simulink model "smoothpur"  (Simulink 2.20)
settings: Solver=ode45  StartTime=0  StopTime=5.0  MaxStep=.01  RelTol=1e-3  AbsTol=1e-3
undefined symbols (not defined in the file or in its folder): sfuny

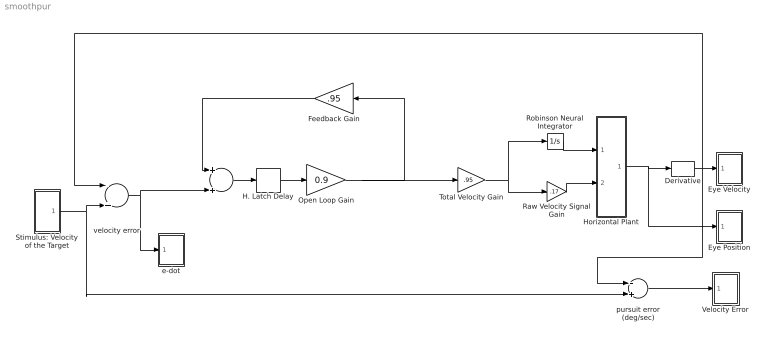
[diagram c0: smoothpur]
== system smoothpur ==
  "  " : Sum  Inputs=++
  Derivative : Derivative
  Eye Position : Subsystem  LoadFcn=sfuny([],[],[],'LoadBlock')  StartFcn=sfuny([],[],[],'Start')  StopFcn=sfuny([],[],[],'Stop')  mask(Graph scope.){}
      mask help: Graph scope using MATLAB graph window. Enter plotting ranges and line type.
      mask init:
      | color = @4; ax = [0, @1, @2, @3]; dt = -1;
  Eye Velocity : Subsystem  LoadFcn=sfuny([],[],[],'LoadBlock')  StartFcn=sfuny([],[],[],'Start')  StopFcn=sfuny([],[],[],'Stop')  mask(Graph scope.){}
      mask help: Graph scope using MATLAB graph window. Enter plotting ranges and line type.
      mask init:
      | color = @4; ax = [0, @1, @2, @3]; dt = -1;
  Feedback Gain : Gain  Orientation=left  Gain=.95
  H. Latch Delay : TransportDelay  DelayTime=.07  InitialInput=00  BufferSize=1024
  Horizontal Plant : Subsystem
  Open Loop Gain : Gain  Gain=0.9
  Raw Velocity Signal Gain : Gain  Gain=.17
  Robinson Neural Integrator : Integrator  ExternalReset=none  InitialConditionSource=internal  InitialCondition=0  LimitOutput=off  UpperSaturationLimit=inf  LowerSaturationLimit=-inf  ShowSaturationPort=off  ShowStatePort=off  AbsoluteTolerance=auto
  Stimulus: Velocity of the Target : Subsystem
  Total Velocity Gain : Gain  Gain=.95
  Velocity Error : Subsystem  LoadFcn=sfuny([],[],[],'LoadBlock')  StartFcn=sfuny([],[],[],'Start')  StopFcn=sfuny([],[],[],'Stop')  mask(Graph scope.){}
      mask help: Graph scope using MATLAB graph window. Enter plotting ranges and line type.
      mask init:
      | color = @4; ax = [0, @1, @2, @3]; dt = -1;
  e-dot : Subsystem  LoadFcn=sfuny([],[],[],'LoadBlock')  StartFcn=sfuny([],[],[],'Start')  StopFcn=sfuny([],[],[],'Stop')  mask(Graph scope.){}
      mask help: Graph scope using MATLAB graph window. Enter plotting ranges and line type.
      mask init:
      | color = @4; ax = [0, @1, @2, @3]; dt = -1;
  pursuit error (deg/sec) : Sum  Inputs=-+
  velocity error : Sum  Inputs=-+
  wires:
  Raw Velocity Signal Gain/1 -> Horizontal Plant/2(in_2)
  Robinson Neural Integrator/1 -> Horizontal Plant/1(in_1)
  Horizontal Plant/1(out_1) -> Derivative/1, Eye Position/1(x)
  Feedback Gain/1 -> "  "/1
  Stimulus: Velocity of the Target/1(out_1) -> velocity error/2, pursuit error (deg/sec)/2
  pursuit error (deg/sec)/1 -> Velocity Error/1(x)
  Derivative/1 -> pursuit error (deg/sec)/1, Eye Velocity/1(x), velocity error/1
  Open Loop Gain/1 -> Feedback Gain/1, Total Velocity Gain/1
  Total Velocity Gain/1 -> Robinson Neural Integrator/1, Raw Velocity Signal Gain/1
  "  "/1 -> H. Latch Delay/1
  H. Latch Delay/1 -> Open Loop Gain/1
  velocity error/1 -> e-dot/1(x), "  "/2

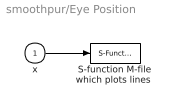
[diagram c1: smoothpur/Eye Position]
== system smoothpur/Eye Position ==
  x : Inport  Port=1  PortWidth=-1  SampleTime=-1
  "S-function M-file which plots lines " : S-Function  FunctionName=sfuny  Parameters=ax, color,dt  PortCounts=[]  SFunctionModules=''
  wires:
  x/1 -> "S-function M-file which plots lines "/1

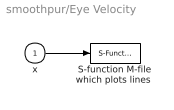
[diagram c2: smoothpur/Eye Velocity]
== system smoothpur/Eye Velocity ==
  x : Inport  Port=1  PortWidth=-1  SampleTime=-1
  "S-function M-file which plots lines " : S-Function  FunctionName=sfuny  Parameters=ax, color,dt  PortCounts=[]  SFunctionModules=''
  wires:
  x/1 -> "S-function M-file which plots lines "/1

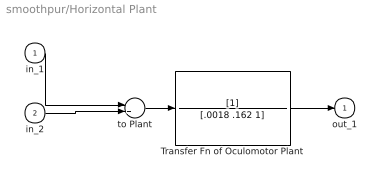
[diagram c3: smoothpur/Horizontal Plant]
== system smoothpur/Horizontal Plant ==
  in_1 : Inport  Port=1  PortWidth=-1  SampleTime=-1
  in_2 : Inport  Port=2  PortWidth=-1  SampleTime=-1
  Transfer Fn of Oculomotor Plant : TransferFcn  Numerator=[1]  Denominator=[.0018 .162 1]
  to Plant : Sum  Inputs=++
  out_1 : Outport  Port=1  InitialOutput=0
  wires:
  Transfer Fn of Oculomotor Plant/1 -> out_1/1
  in_2/1 -> to Plant/2
  in_1/1 -> to Plant/1
  to Plant/1 -> Transfer Fn of Oculomotor Plant/1

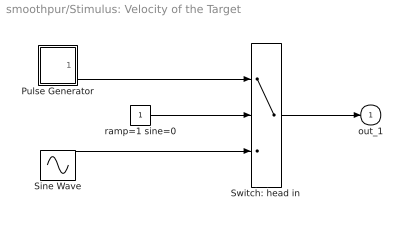
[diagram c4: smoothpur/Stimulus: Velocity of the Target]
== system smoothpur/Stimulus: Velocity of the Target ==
  Pulse Generator : Subsystem  mask(Pulse Generator){}
      mask help: Pulse Generator.
      mask init:
      | Ts=@1; du=@2; ht=@3; stt=@4; ini=ones(length(ht),1); st1=rem(stt,Ts); st2=rem(stt+du,Ts);if(Ts<=1.2*du),ini=zeros(length(ht),1);end;
  Sine Wave : Sin  Amplitude=10  Frequency=1*pi*2  Phase=0  SampleTime=-1
  Switch: head in : Switch  Threshold=.5
  ramp=1 sine=0 : Constant  Value=1
  out_1 : Outport  Port=1  InitialOutput=0
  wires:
  Sine Wave/1 -> Switch: head in/3
  Pulse Generator/1(out_1) -> Switch: head in/1
  Switch: head in/1 -> out_1/1
  ramp=1 sine=0/1 -> Switch: head in/2

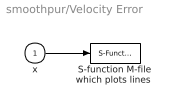
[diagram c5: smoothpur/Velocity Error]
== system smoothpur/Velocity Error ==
  x : Inport  Port=1  PortWidth=-1  SampleTime=-1
  "S-function M-file which plots lines " : S-Function  FunctionName=sfuny  Parameters=ax, color,dt  PortCounts=[]  SFunctionModules=''
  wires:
  x/1 -> "S-function M-file which plots lines "/1

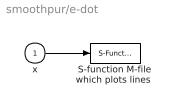
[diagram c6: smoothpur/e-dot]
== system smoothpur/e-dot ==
  x : Inport  Port=1  PortWidth=-1  SampleTime=-1
  "S-function M-file which plots lines " : S-Function  FunctionName=sfuny  Parameters=ax, color,dt  PortCounts=[]  SFunctionModules=''
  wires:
  x/1 -> "S-function M-file which plots lines "/1

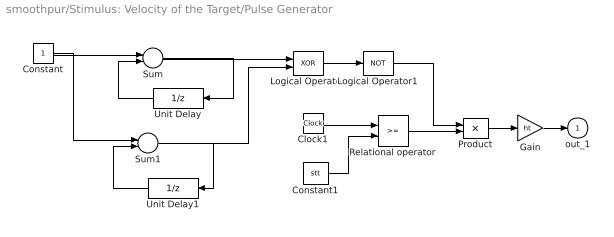
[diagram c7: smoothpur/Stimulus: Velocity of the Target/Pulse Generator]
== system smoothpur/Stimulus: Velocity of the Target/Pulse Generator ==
  Clock1 : Clock
  Constant : Constant  Value=1
  Constant1 : Constant  Value=stt
  Gain : Gain  Gain=ht
  Logical Operator : Logic  Operator=XOR  Inputs=2
  Logical Operator1 : Logic  Operator=NOT  Inputs=1
  Product : Product  Inputs=2
  Relational operator : RelationalOperator  Operator=>=
  Sum : Sum  Inputs=+-
  Sum1 : Sum  Inputs=+-
  Unit Delay : UnitDelay  Orientation=left  X0=0  SampleTime=[Ts,st1]
  Unit Delay1 : UnitDelay  Orientation=left  X0=ini  SampleTime=[Ts,st2]
  out_1 : Outport  Port=1  InitialOutput=0
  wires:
  Sum1/1 -> Logical Operator/2, Unit Delay1/1
  Sum/1 -> Logical Operator/1, Unit Delay/1
  Constant/1 -> Sum1/1, Sum/1
  Unit Delay1/1 -> Sum1/2
  Unit Delay/1 -> Sum/2
  Clock1/1 -> Relational operator/1
  Relational operator/1 -> Product/2
  Product/1 -> Gain/1
  Gain/1 -> out_1/1
  Constant1/1 -> Relational operator/2
  Logical Operator/1 -> Logical Operator1/1
  Logical Operator1/1 -> Product/1
